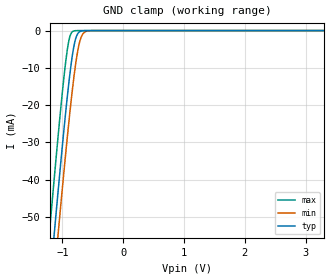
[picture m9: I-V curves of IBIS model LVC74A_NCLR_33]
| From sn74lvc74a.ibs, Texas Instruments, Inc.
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[Model]   LVC74A_NCLR_33
Model_type  Input
Vinl=0.8
Vinh=2.0
| variable   typ   min   max
C_comp   4.71pF   3.65pF   6.00pF
[Temperature Range]   40   100   -40
| Ambient temperature   25   85   -40
[Voltage range]   3.3   3   3.6
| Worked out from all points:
|   GND clamp passes 1 mA (typ) near -0.75 V on its own axis
[GND Clamp]
| LVC74A_NCLR_33
|   Voltage   I(typ)   I(min)   I(max)
-5.5V     -915.9mA   -925.7mA   -903.9mA
-1.225V   -71.19mA   -82.77mA   -56.33mA
-1.145V   -56.44mA   -68.03mA   -41.55mA
-1.12V    -51.89mA   -63.47mA   -37.02mA
-1.08V    -44.71mA   -56.26mA   -29.89mA
-1.06V    -41.16mA   -52.69mA   -26.4mA
-965mV    -24.94mA   -36.16mA   -11.03mA
-885mV    -12.72mA   -23.13mA   -2.077mA
-780mV    -2.057mA   -8.704mA   -23.97uA
-715mV    -287.1uA   -2.975mA   -1.13uA
-640mV    -21.7uA    -472.6uA   -33.12nA
3.3V      11.73pA    10.22pA    5.93pA
